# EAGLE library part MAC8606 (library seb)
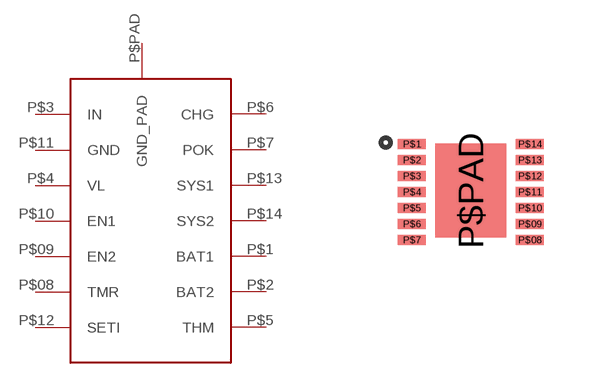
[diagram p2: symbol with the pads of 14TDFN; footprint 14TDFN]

Designator prefix IC

## MAC8606  [14TDFN]
P$1  BAT1
P$2  BAT2
P$3  IN
P$4  VL
P$5  THM
P$6  CHG
P$7  POK
P$08  TMR
P$09  EN2
P$10  EN1
P$11  GND
P$12  SETI
P$13  SYS1
P$14  SYS2
P$PAD  GND_PAD

## Footprint 14TDFN (pad centres in mm)
smd 0.7 x 0.25: P$1 -1.35,1.05; P$2 -1.35,0.65; P$3 -1.35,0.25; P$4 -1.35,-0.15; P$5 -1.35,-0.55; P$6 -1.35,-0.95; P$7 -1.35,-1.35; P$08 1.6,-1.35; P$09 1.6,-0.95; P$10 1.6,-0.55; P$11 1.6,-0.15; P$12 1.6,0.25; P$13 1.6,0.65; P$14 1.6,1.05
smd 1.78 x 2.35: P$PAD 0.12,-0.12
